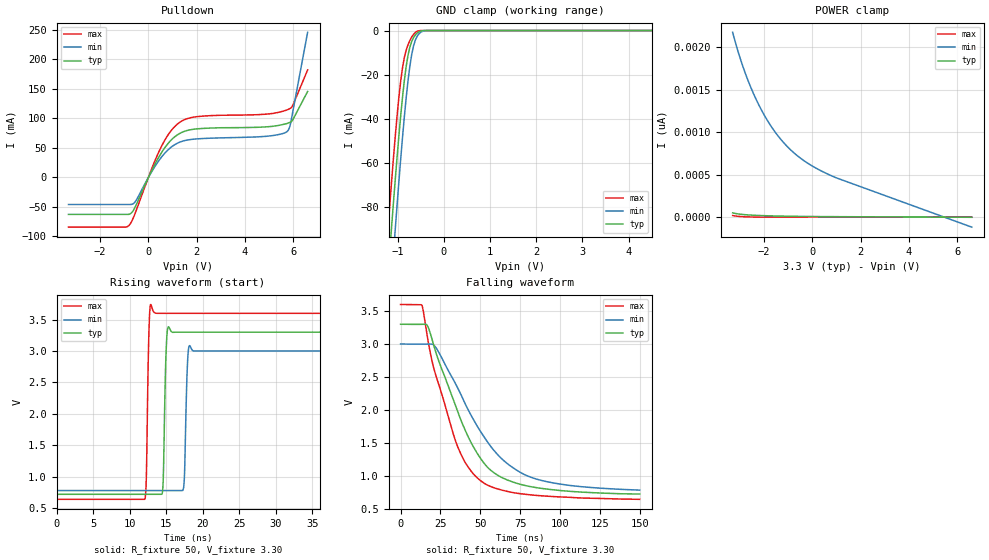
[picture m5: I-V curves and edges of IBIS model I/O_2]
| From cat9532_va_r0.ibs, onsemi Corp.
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|//////////////////////////////////////////////////////////////////////////////
|//////////////////////////////////////////////////////////////////////////////
[Model] I/O_2
Model_type I/O_open_drain
Enable Active-Low
Polarity Non-Inverting
Vinh = 2.0
Vinl = 0.8
Vref = 3.3V
Vmeas = 1.65
Rref = 50
Cref = 400pF
|  variable   typ   min   max
C_comp   3.018pF   3.018pF   3.018pF
|//////////////////////////////////////////////////////////////////////////////
[Temperature Range]   25   85   -40
|//////////////////////////////////////////////////////////////////////////////
[Voltage Range]   3.30V   3.0V   3.60V
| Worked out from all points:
|   slope of the pulldown table from 0 to 0.495 V, typ, clamps not added: 12.7 ohm
|   GND clamp passes 1 mA (typ) near -0.57 V on its own axis
|   falling waveform, R_fixture 50, V_fixture 3.30: 20-80 % time 27.6ns typ, 34.1ns min, 22.3ns max; typ from 3.3 V to 0.72 V
|   rising waveform, R_fixture 50, V_fixture 3.30: 20-80 % time 272ps typ, 277ps min, 249ps max; typ from 0.72 V to 3.3 V
|//////////////////////////////////////////////////////////////////////////////
[Pulldown]
|   Voltage   I(typ)   I(min)   I(max)
-3.3V     -62.8mA    -46.02mA   -84.4mA
-800mV    -62.68mA   -46.02mA   -81.8mA
-540mV    -50.38mA   -41.45mA   -60.9mA
180mV     14.3mA     11.85mA    18.11mA
600mV     44.93mA    36.76mA    56.37mA
1.02V     65.85mA    53.19mA    82.5mA
1.44V     76.95mA    61.43mA    96.37mA
2.18V     82.58mA    65.52mA    103.4mA
4.9V      85.47mA    69.5mA     107mA
5.74V     91.11mA    77.17mA    114mA
5.9V      93.74mA    92.17mA    117.3mA
6.6V      145.4mA    245.6mA    181.9mA
|//////////////////////////////////////////////////////////////////////////////
[GND Clamp]
|   Voltage   I(typ)   I(min)   I(max)
-3.3V     -698.8mA   -702.5mA   -696.6mA
-1.22V    -112.9mA   -135.2mA   -92.07mA
-1.14V    -90.36mA   -113.4mA   -69.67mA
-1.06V    -68.67mA   -91.31mA   -49mA
-940mV    -39.11mA   -58.77mA   -23.24mA
-900mV    -30.52mA   -48.77mA   -17.02mA
-820mV    -16.37mA   -30.67mA   -8.945mA
-780mV    -11.27mA   -22.89mA   -6.495mA
-700mV    -5.005mA   -10.94mA   -2.971mA
-580mV    -1.094mA   -2.536mA   -344.3uA
-340mV    -852.2nA   -12.85uA   -12.29nA
6.6V      10.57pA    936.5pA    409.9fA
|//////////////////////////////////////////////////////////////////////////////
[POWER Clamp]
|   Voltage   I(typ)   I(min)   I(max)
-3.3V     50.01pA    2.174nA    18.36pA
-3.06V    37.07pA    1.933nA    8.979pA
-2.76V    27.92pA    1.679nA    3.29pA
-2.46V    22.4pA     1.467nA    1.165pA
-2.16V    18.53pA    1.288nA    496.4fA
-1.8V     15.23pA    1.109nA    361fA
-1.44V    12.72pA    962.2pA    346.3fA
-1.08V    10.78pA    842.2pA    331.6fA
-660mV    8.882pA    731pA      314.5fA
60mV      6.764pA    590.5pA    285.1fA
960mV     5.158pA    465.7pA    248.4fA
6.6V      -2.016pA   -118.2pA   18.29fA
|//////////////////////////////////////////////////////////////////////////////
|//////////////////////////////////////////////////////////////////////////////
[Ramp]
|  variable   typ   min   max
dV/dt_r   1.548E+00/2.500E-10  1.332E+00/2.500E-10  1.776E+00/2.500E-10
dV/dt_f   1.548E+00/2.625E-08  1.332E+00/3.375E-08  1.776E+00/2.250E-08
R_load = 50
|//////////////////////////////////////////////////////////////////////////////
[Falling Waveform]
R_fixture = 50
V_fixture = 3.30
V_fixture_min = 3.0
V_fixture_max = 3.60
C_fixture = 0p
|   time   V(typ)   V(min)   V(max)
0s        3.3V       3V         3.6V
13.5ns    3.299V     2.998V     3.588V
16.5ns    3.293V     2.999V     3.158V
20.25ns   3.028V     2.994V     2.688V
33.75ns   2.112V     2.429V     1.581V
40.5ns    1.692V     2.093V     1.202V
49.5ns    1.286V     1.696V     936.7mV
63ns      977.7mV    1.267V     783.7mV
81ns      835.5mV    982.6mV    709.1mV
150ns     720mV      780mV      640mV
|//////////////////////////////////////////////////////////////////////////////
[Rising Waveform]
R_fixture = 50
V_fixture = 3.30
V_fixture_min = 3.0
V_fixture_max = 3.60
C_fixture = 0p
|   time   V(typ)   V(min)   V(max)
0s        720mV      780mV      640mV
12.1ns    720mV      780mV      645.2mV
12.65ns   720mV      780mV      3.326V
12.9ns    720mV      780mV      3.741V
14.5ns    756mV      780mV      3.6V
14.95ns   2.843V     780mV      3.6V
15.3ns    3.387V     780mV      3.6V
17.4ns    3.3V       829.6mV    3.6V
18.2ns    3.3V       3.086V     3.6V
150ns     3.3V       3V         3.6V
